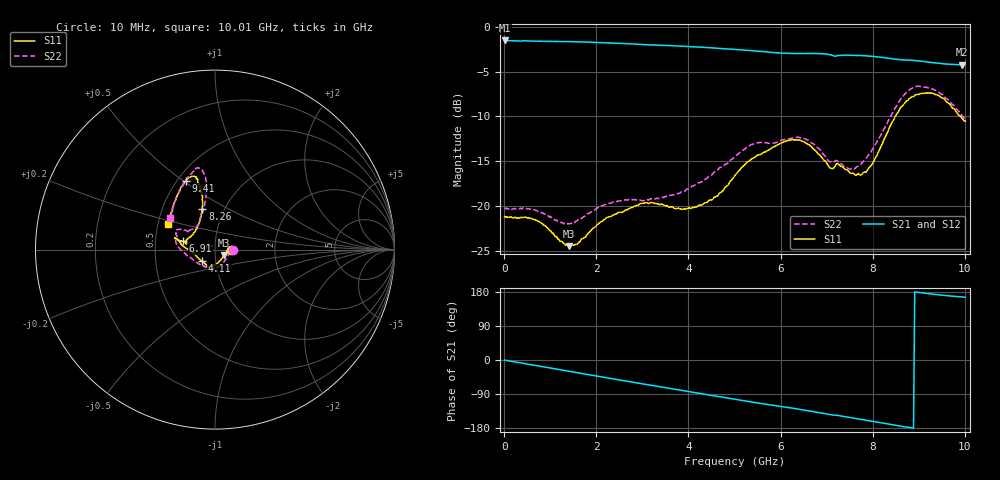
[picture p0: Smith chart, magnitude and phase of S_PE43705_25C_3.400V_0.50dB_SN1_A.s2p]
! Device ID: PE43705
! Serial: 1
! Insertion: A
! Impedance: 50 ohm
! Temp: 25C
! VDD: 3.400V
! Attenuation Step: 0.50dB
#  Hz  S  RI  R  50
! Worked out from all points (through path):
!   401 points, 10 MHz to 10.01 GHz, reference 50 ohm
!   highest |S21| = -1.50 dB at 10 MHz (marker M1); lowest = -4.2 dB at 9.935 GHz (marker M2)
!   group delay of S21, straight-line fit = 55.2 ps
!   lowest |S11| = -24.5 dB at 1.41 GHz (marker M3), VSWR 1.13, Z = 55.2 - j3.5 ohm
!   |S11| at or under -10 dB: start of sweep to 8.487 GHz; 9.903 GHz to end of sweep
!   |S22| runs from -22.0 to -6.6 dB; largest |S21 - S12| = 0.0074
!   S11 on the Smith chart (normalised r, x): 10 MHz: 1.19, -0.00; 4.11 GHz: 0.86, -0.11; 6.91 GHz: 0.69, +0.07; 8.26 GHz: 0.79, +0.38; 9.41 GHz: 0.55, +0.51; 10.01 GHz: 0.57, +0.18
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1e7  0.0874 -0.000764  0.8409 -0.00434  0.8413 -0.004  0.0977 -0.000736
7.1e8  0.0823 0.0124  0.8052 -0.216  0.8053 -0.2158  0.0942 0.00448
1.41e9  0.0505 -0.0315  0.7191 -0.4112  0.7193 -0.411  0.0639 -0.0471
1.685e9  0.0337 -0.0561  0.6713 -0.4798  0.6712 -0.4801  0.0437 -0.0736
2.235e9  7.07e-05 -0.0862  0.5551 -0.5975  0.5554 -0.597  -0.00103 -0.1031
3.36e9  -0.0399 -0.0942  0.2686 -0.744  0.2696 -0.7434  -0.058 -0.0939
4.11e9  -0.0737 -0.0643  0.0613 -0.7731  0.0626 -0.7728  -0.1123 -0.0648
4.585e9  -0.107 -0.0341  -0.0679 -0.7597  -0.0671 -0.7594  -0.1512 -0.0376
5.01e9  -0.1479 0.000909  -0.1769 -0.7277  -0.1761 -0.7279  -0.1892 -0.00216
5.41e9  -0.1842 0.0238  -0.27 -0.6844  -0.2694 -0.685  -0.218 0.0402
6.11e9  -0.2203 0.0644  -0.4028 -0.5879  -0.3991 -0.5885  -0.2156 0.0919
6.685e9  -0.2047 0.053  -0.5076 -0.4974  -0.5078 -0.4966  -0.1934 0.1132
6.91e9  -0.1786 0.046  -0.5464 -0.4511  -0.547 -0.4517  -0.1645 0.1081
7.46e9  -0.1416 0.0695  -0.6078 -0.3397  -0.6061 -0.3403  -0.1126 0.1169
7.76e9  -0.1094 0.1027  -0.6367 -0.2688  -0.6355 -0.2713  -0.0926 0.1467
7.985e9  -0.0892 0.1464  -0.6514 -0.2145  -0.6508 -0.2178  -0.0756 0.1912
8.26e9  -0.0706 0.2289  -0.6571 -0.1467  -0.655 -0.1523  -0.0542 0.2677
8.36e9  -0.0689 0.2646  -0.657 -0.1227  -0.6559 -0.126  -0.0501 0.3043
8.86e9  -0.1046 0.3946  -0.6511 -0.00721  -0.6471 -0.0118  -0.0827 0.448
9.41e9  -0.1633 0.3824  -0.6222 0.0853  -0.62 0.0842  -0.1443 0.4146
9.935e9  -0.252 0.1799  -0.598 0.1439  -0.6004 0.1449  -0.24 0.2117
1.001e10  -0.2612 0.1428  -0.5987 0.1528  -0.6014 0.1513  -0.251 0.1763
